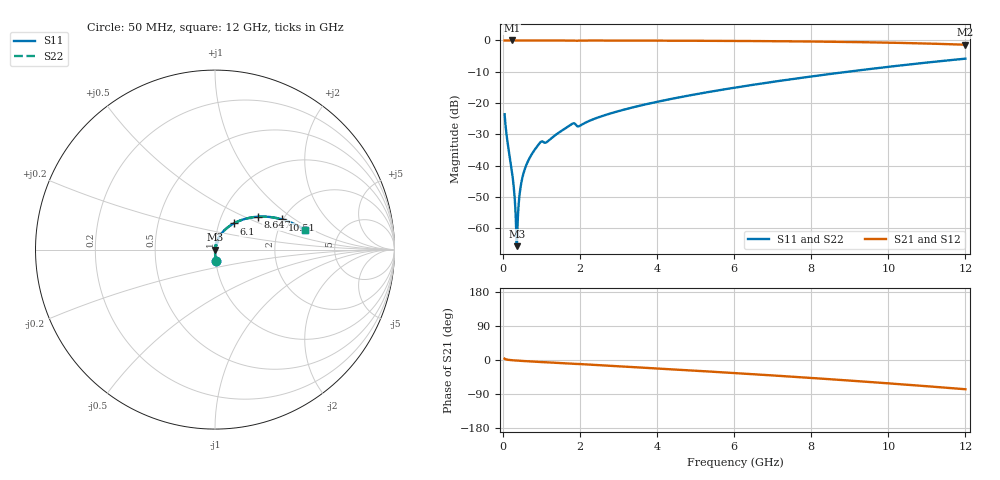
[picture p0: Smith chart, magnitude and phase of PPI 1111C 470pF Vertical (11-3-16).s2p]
# GHz S MA R 50
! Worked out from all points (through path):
!   1601 points, 50 MHz to 12 GHz, reference 50 ohm
!   highest |S21| = 0.00 dB at 236.7 MHz (marker M1); lowest = -1.4 dB at 12 GHz (marker M2)
!   group delay of S21, straight-line fit = 17.7 ps
!   lowest |S11| = -65.8 dB at 363.7 MHz (marker M3), VSWR 1.00, Z = 50.1 - j0.0109 ohm
!   |S11| at or under -10 dB: start of sweep to 8.95 GHz
!   |S22| runs from -65.8 to -5.8 dB; largest |S21 - S12| = 0
!   S11 on the Smith chart (normalised r, x): 50 MHz: 1.00, -0.13; 6.1 GHz: 1.18, +0.35; 8.647 GHz: 1.48, +0.59; 10.51 GHz: 1.98, +0.80; 12 GHz: 2.81, +0.84
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0.05  0.06625 -86.2  0.9975 3.6  0.9975 3.6  0.06625 -86.2
0.2367188  0.008327 -87.6  0.9995 -0.5  0.9995 -0.5  0.008327 -87.6
0.2740625  0.005441 -86.1  0.9995 -0.8  0.9995 -0.8  0.005441 -86.1
0.3263437  0.002169 -78.3  0.9995 -1.2  0.9995 -1.2  0.002169 -78.3
0.3636875  0.0005156 -12.2  0.9995 -1.5  0.9995 -1.5  0.0005156 -12.2
0.4010313  0.001807 71.3  0.9994 -1.8  0.9994 -1.8  0.001807 71.3
0.46825  0.004709 80.9  0.9994 -2.2  0.9994 -2.2  0.004709 80.9
0.5429375  0.007646 82.8  0.9993 -2.7  0.9993 -2.7  0.007646 82.8
0.6624375  0.01198 83.2  0.9992 -3.4  0.9992 -3.4  0.01198 83.2
0.8491562  0.0186 82.0  0.9987 -4.6  0.9987 -4.6  0.0186 82.0
0.9835938  0.02374 76.7  0.9964 -5.4  0.9964 -5.4  0.02374 76.7
1.147906  0.02385 76.1  0.9964 -6.1  0.9964 -6.1  0.02385 76.1
1.790219  0.04604 74.6  0.9945 -10.0  0.9945 -10.0  0.04604 74.6
2.044156  0.04483 74.5  0.9954 -11.0  0.9954 -11.0  0.04483 74.5
4.038312  0.1056 66.5  0.9925 -22.6  0.9925 -22.6  0.1056 66.5
6.025  0.1762 54.8  0.982 -34.5  0.982 -34.5  0.1762 54.8
6.099687  0.1792 54.3  0.9814 -35.0  0.9814 -35.0  0.1792 54.3
8.019156  0.2664 42.0  0.9609 -47.5  0.9609 -47.5  0.2664 42.0
8.646531  0.2994 37.7  0.951 -51.8  0.951 -51.8  0.2994 37.7
10.01331  0.3793 27.9  0.9216 -61.7  0.9216 -61.7  0.3793 27.9
10.50625  0.4106 24.2  0.908 -65.4  0.908 -65.4  0.4106 24.2
12  0.5116 12.4  0.8548 -77.2  0.8548 -77.2  0.5116 12.4
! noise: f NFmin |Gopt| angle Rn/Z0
0.05  0.0003434  0.8556  0.2534  0.0005082
1.372  0.004539  0.7224  5.575  0.003235
2.701  0.006365  0.6325  10.72  0.003229
4.031  0.008102  0.5855  15.6  0.003506
5.36  0.01002  0.5655  20.32  0.004036
6.682  0.01199  0.557  24.82  0.004644
8.012  0.01408  0.5567  29.17  0.005361
9.341  0.01634  0.5633  33.37  0.006224
10.67  0.01886  0.5758  37.46  0.007293
12  0.0217  0.5937  41.47  0.008651
